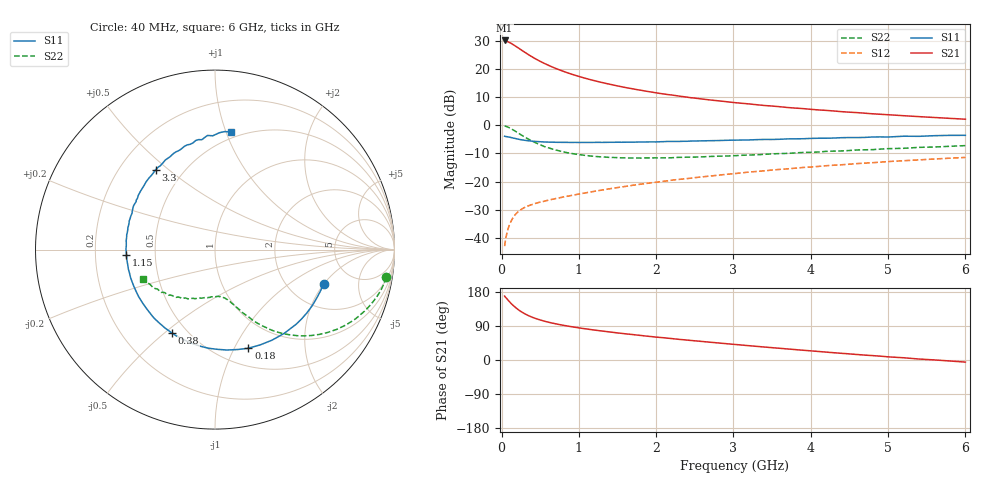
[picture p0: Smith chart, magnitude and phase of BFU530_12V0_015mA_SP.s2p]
! Filename:  P:\Prog\Test\Noise\ATS_data\Testdata_Net\03 Spar\BFU530_APG2013_40_A05_12p0V_015mA_SP_CM01_D.s2p
! Date/Time: Fri 26/Apr/2013 13:03:12
! BFU530_APG2013_40_A05_12p0V_1to25mA_SP_CM01_Bias6_R.s2p
! MDIF S-parameter v. bias file
! BFU530_APG2013_40_A05_12p0V_1to25mA_SP_CM01
! Date/time Wed Apr 24 20:41:12 2013
! VAR V_out= 12.0010
! VAR I_out= 15.0050
! VAR V_in= 0.7980
! VAR I_in= 0.1454
! Device data file deembeded for feedlines and parallel
! Original file: \03 Spar\BFU530_APG2013_40_A05_12p0V_015mA_SP_CM01_R.s2p
! Feed-files: PR047V01_250413_Feed1.s2p, PR047V01_250413_Feed2.s2p
! Parallel-file: PR047V01_250413_Par.s2p
# MHz S MA R 50
!  Freq-MHz  S11-mag  S11-arg  S21-mag  S21-arg  S12-mag  S12-arg  S22-mag  S22-arg
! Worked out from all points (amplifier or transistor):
!   98 points, 40 MHz to 6 GHz, reference 50 ohm
!   highest |S21| = 30.1 dB at 40 MHz (marker M1)
!   |S21| within 3 dB of that: start of sweep to 235.5 MHz
!   unconditionally stable (mu >= 1): 1.573 GHz to 3.84 GHz
!   at 300 MHz: K = 0.38, MSG = 27.6 dB, |S12| = -29.2 dB
!   at 1.6 GHz: K = 1.01, MAG = 17.1 dB, |S12| = -21.7 dB
!   at 6 GHz: K = 0.88, MSG = 6.8 dB, |S12| = -11.4 dB
!   S11 on the Smith chart (normalised r, x): 40 MHz: 3.11, -2.00; 180 MHz: 0.69, -1.14; 380 MHz: 0.41, -0.53; 1.15 GHz: 0.34, -0.03; 3.3 GHz: 0.35, +0.45; 6 GHz: 0.45, +1.04
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40  0.6358 -17.5  31.93 168.8  0.007117 80.3  0.9665 -9.2
50  0.6307 -22.0  31.81 165.7  0.008852 78.6  0.9596 -11.6
90  0.6181 -38.7  29.91 156.7  0.01516 72.5  0.9143 -20.4
120  0.6052 -50.6  28.59 150.1  0.01933 68.2  0.8719 -26.4
140  0.5962 -57.9  27.53 146.0  0.02176 65.6  0.8411 -30.0
180  0.58 -71.3  25.39 138.8  0.02609 61.1  0.7793 -36.3
220  0.5634 -83.2  23.39 132.3  0.02948 57.6  0.7199 -41.7
280  0.5452 -98.0  20.55 124.4  0.03351 53.8  0.6396 -48.1
320  0.5345 -106.6  18.96 119.9  0.03571 52.0  0.5949 -51.6
380  0.5232 -117.3  16.82 114.3  0.03846 50.2  0.5358 -55.8
500  0.5087 -133.6  13.61 105.7  0.04311 48.6  0.4497 -61.7
650  0.4997 -148.3  10.9 97.7  0.04813 48.6  0.3801 -66.7
800  0.4957 -158.8  9.035 91.6  0.0531 49.5  0.3365 -70.2
1050  0.494 -172.5  7.015 83.3  0.0616 51.1  0.2948 -75.1
1150  0.494 -176.7  6.431 80.5  0.06517 51.7  0.284 -76.7
1600  0.4985 167.1  4.671 69.2  0.0818 53.1  0.2632 -84.4
2050  0.5083 155.2  3.661 59.6  0.09892 53.1  0.2631 -92.3
3100  0.5443 130.8  2.453 39.6  0.1422 50.0  0.2918 -111.0
3300  0.5539 126.8  2.309 36.0  0.1509 48.9  0.2981 -114.3
4100  0.5865 111.7  1.866 22.5  0.1855 43.9  0.3342 -127.8
5200  0.6373 93.8  1.474 5.9  0.2341 35.5  0.3885 -145.5
6000  0.6606 82.5  1.277 -5.5  0.2677 28.4  0.4339 -157.8
